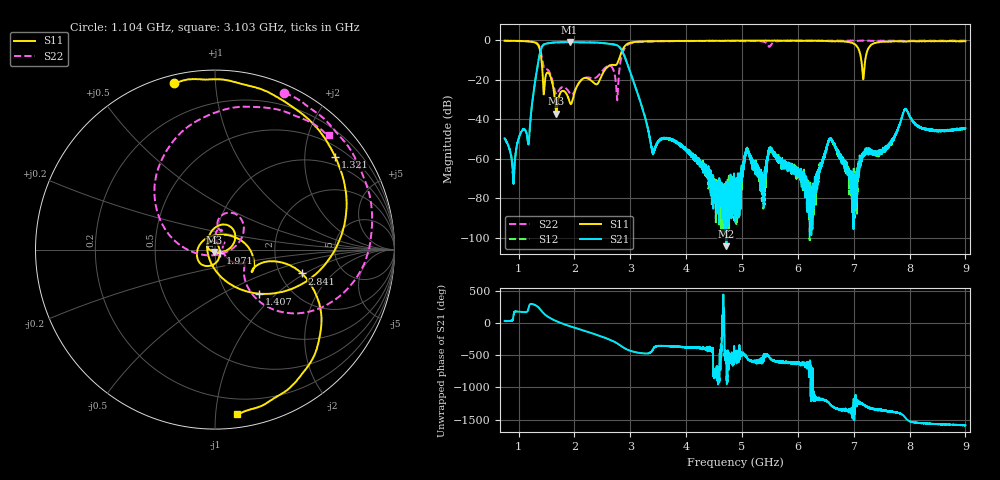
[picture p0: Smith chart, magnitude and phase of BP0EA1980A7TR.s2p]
!Agilent Technologies,E8358A,US41080443,A.07.50.56
!Agilent E8358A: A.07.50.56
!Date: Friday, November 20, 2015 11:03:19
!Correction: S11(Full 2 Port(1,2))
!S21(Full 2 Port(1,2))
!S12(Full 2 Port(1,2))
!S22(Full 2 Port(1,2))
!S2P File: Measurements: S11, S21, S12, S22:
# Hz S  dB  R 50
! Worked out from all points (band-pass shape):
!   6401 points, 750 MHz to 9 GHz, reference 50 ohm
!   highest |S21| = -0.81 dB at 1.913 GHz (marker M1); lowest = -104.3 dB at 4.722 GHz (marker M2)
!   |S21| within 3 dB of the highest: 1.408 GHz to 2.822 GHz (1.414 GHz wide, 66.8 % of centre)
!   lowest |S11| = -37.1 dB at 1.676 GHz (marker M3), VSWR 1.03, Z = 49.6 - j1.33 ohm
!   |S11| at or under -10 dB: 1.411 GHz to 2.792 GHz (1.381 GHz wide, 65.7 % of centre); 7.137 GHz to 7.207 GHz (69.84 MHz wide, 0.974 % of centre)
!   |S22| runs from -30.3 to 0.0 dB; largest |S21 - S12| = 0.0062
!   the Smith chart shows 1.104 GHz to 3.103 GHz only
!   S11 on the Smith chart (normalised r, x): 1.104 GHz: 0.03, +0.79; 1.321 GHz: 0.76, +2.76; 1.407 GHz: 1.40, -0.78; 1.971 GHz: 1.05, -0.04; 2.841 GHz: 2.64, -0.94; 3.103 GHz: 0.09, -1.14
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7.5e8  -0.11 142.4  -49.65 38.7  -49.71 38.7  -0.21 114.3
1.104492e9  -0.37 103.7  -45.10 174.5  -45.15 174.5  -0.40 66.1
1.321055e9  -1.45 37.5  -16.20 -85.7  -16.23 -85.6  -1.16 5.4
1.407422e9  -9.20 -45.1  -3.89 -161.5  -3.93 -161.5  -6.90 -46.5
1.675547e9  -37.10 -105.7  -0.95 35.4  -0.98 35.4  -27.25 3.1
1.912734e9  -31.06 50.1  -0.81 -42.6  -0.86 -42.6  -26.49 41.6
1.970742e9  -29.76 -34.7  -0.81 -59.4  -0.85 -59.4  -27.18 68.1
2.12543e9  -19.91 -114.4  -0.87 -102.2  -0.91 -102.2  -20.08 85.9
2.439961e9  -20.83 66.3  -1.14 169.5  -1.17 169.5  -17.41 83.9
2.840859e9  -5.98 -15.3  -4.55 4.2  -4.63 4.2  -8.52 147.9
3.102539e9  -0.67 -82.4  -24.44 -91.2  -24.53 -91.1  -0.94 45.1
3.500859e9  -0.34 -124.0  -51.19 7.3  -51.04 8.1  -0.40 -11.0
4.721602e9  -0.19 -177.7  -104.28 160.3  -77.54 -125.6  -0.19 -98.9
4.875e9  -0.12 178.7  -85.25 -89.2  -74.10 -179.4  -0.20 -107.3
5.514375e9  -0.13 -174.0  -55.57 168.4  -55.11 166.5  -2.52 -141.0
6.25043e9  -0.10 -176.5  -75.95 44.1  -87.37 -62.7  -0.15 -174.6
6.576562e9  -0.34 178.5  -49.86 179.5  -49.89 -179.3  -0.18 175.5
7.009688e9  -1.76 147.9  -71.59 -70.5  -86.07 104.2  -0.16 166.0
7.175977e9  -19.09 -22.2  -57.26 170.3  -57.43 169.5  -0.11 163.0
7.625859e9  -0.58 -175.0  -53.59 69.9  -53.50 63.4  -0.18 153.8
7.9275e9  -0.55 168.2  -34.78 -35.8  -34.74 -33.9  -0.26 148.2
9e9  -0.40 126.1  -44.54 -149.7  -44.67 -149.6  -0.11 120.9
